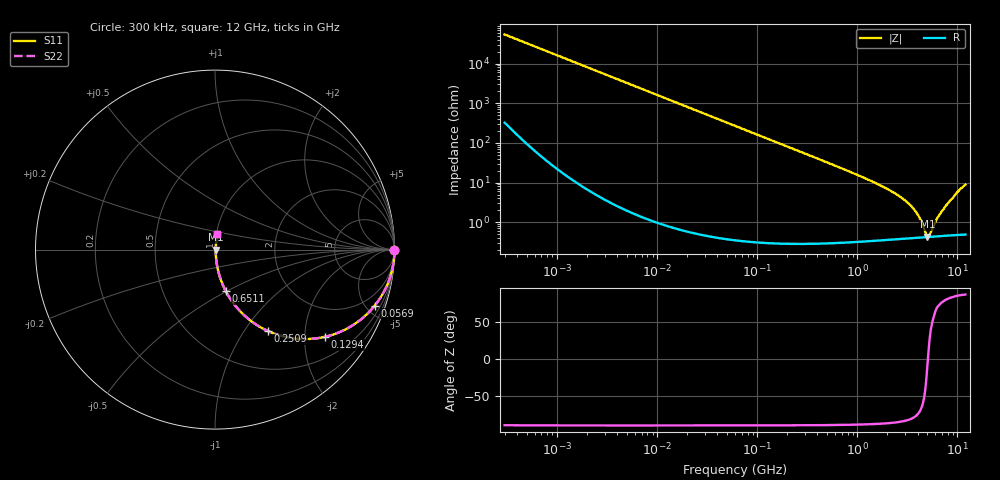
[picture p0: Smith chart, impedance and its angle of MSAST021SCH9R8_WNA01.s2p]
! MSAST021SCH9R8_WNA01  S-PARAMETER MODEL  ( General Type )
! Model Generated by TAIYO YUDEN Corporation (http://www.ty-top.com)
! Version 2.0
! TAIYO YUDEN Control No. 181101
! Copyright(c) 2015 TAIYO YUDEN CO.,LTD. All Rights Reserved.
! Product Description (link to TY-COMPAS)
! https://ds.yuden.co.jp/TYCOMPAS/or/detail?pn=MSAST021SCH9R8CWNA01&u=M
! Products Name : Multilayer Ceramic Capacitors
! Characteristics :
!  Capacitance : 9.8 pF , Rated Voltage : 25V , TCC : CH / C0H
!  Case Size : 0.25 x 0.125 / 0.0098 x 0.0049 [mm/inch] , Thickness : 0.125 / 0.0049 [mm/inch]
!  (Conditions: Temperature = 25 degC , DC Bias Current/Voltage = 0A / 0V)
! External Node Assignments :
!  1  o---| |---o  2
! GND o---------o GND
! Frequency Range : 0.3MHz  -  12000MHz  [ 401 STEP ]
# MHz S RI R 50
! Freq[MHz].  S11 Real  S11 Imag  S21 Real  S21 Imag  S12 Real  S12 Imag  S22 Real  S22 Imag
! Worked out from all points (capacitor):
!   401 points, 300 kHz to 12 GHz, reference 50 ohm
!   read as one part in series: C = 9.8 pF near 316.3 kHz
!   lowest |Z| = 431 mohm at 5.006 GHz (marker M1)
!   series resonance near 5.067 GHz, so ESL is about 100 pH
!   S11 on the Smith chart (normalised r, x): 300 kHz: open; 56.9 MHz: 1.01, -5.71; 129.4 MHz: 1.01, -2.51; 250.9 MHz: 1.01, -1.29; 651.1 MHz: 1.01, -0.49; 12 GHz: 1.01, +0.18
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0.3  1 -0.00185  1.45e-05 0.00185  1.45e-05 0.00185  1 -0.00185
1.769972  0.9999 -0.0109  0.000128 0.0109  0.000128 0.0109  0.9999 -0.0109
10.44266  0.9958 -0.064  0.00416 0.064  0.00416 0.064  0.9958 -0.064
25.70316  0.9754 -0.1544  0.0246 0.1544  0.0246 0.1544  0.9754 -0.1544
56.90376  0.8903 -0.3119  0.1097 0.3119  0.1097 0.3119  0.8903 -0.3119
60  0.8796 -0.3248  0.1204 0.3248  0.1204 0.3248  0.8796 -0.3248
86.94074  0.7768 -0.4156  0.2232 0.4156  0.2232 0.4156  0.7768 -0.4156
129.3602  0.6113 -0.4863  0.3887 0.4863  0.3887 0.4863  0.6113 -0.4863
250.8588  0.2951 -0.4539  0.7049 0.4539  0.7049 0.4539  0.2951 -0.4539
353.9943  0.174 -0.376  0.826 0.376  0.826 0.376  0.174 -0.376
651.0506  0.0593 -0.2301  0.9407 0.2301  0.9407 0.2301  0.0593 -0.2301
2088.533  0.0077 -0.0638  0.9923 0.0638  0.9923 0.0638  0.0077 -0.0638
2870.14  0.00528 -0.038  0.9947 0.038  0.9947 0.038  0.00528 -0.038
3547.679  0.00451 -0.023  0.9955 0.023  0.9955 0.023  0.00451 -0.023
4158.869  0.00426 -0.0125  0.9957 0.0125  0.9957 0.0125  0.00426 -0.0125
4747.894  0.00422 -0.00402  0.9958 0.00402  0.9958 0.00402  0.00422 -0.00402
5006.236  0.00424 -0.00063  0.9958 0.00063  0.9958 0.00063  0.00424 -0.00063
5278.635  0.00429 0.00223  0.9957 -0.00223  0.9957 -0.00223  0.00429 0.00223
6354.153  0.00458 0.0125  0.9954 -0.0125  0.9954 -0.0125  0.00458 0.0125
7254.098  0.00495 0.0207  0.9951 -0.0207  0.9951 -0.0207  0.00495 0.0207
9968.853  0.00791 0.0561  0.9921 -0.0561  0.9921 -0.0561  0.00791 0.0561
12000  0.0125 0.0869  0.9875 -0.0869  0.9875 -0.0869  0.0125 0.0869
